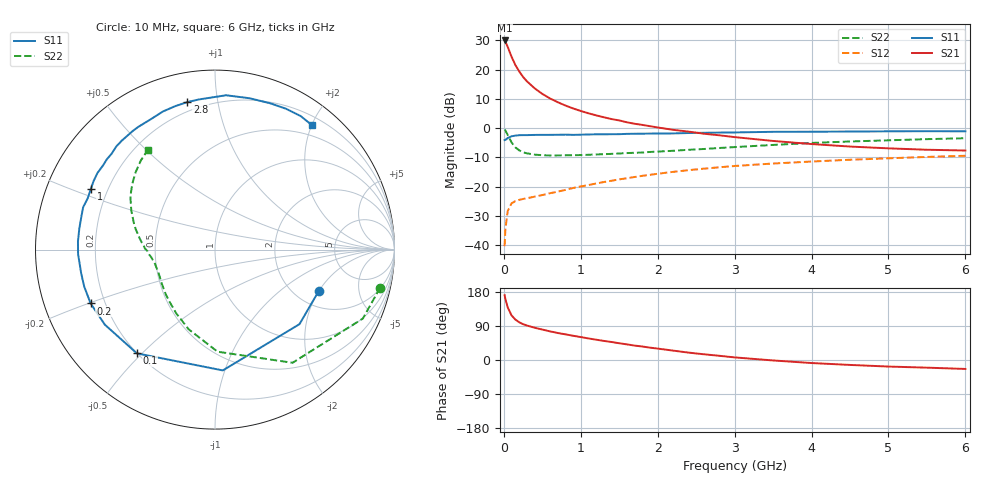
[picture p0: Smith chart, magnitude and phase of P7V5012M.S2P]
! SIEMENS Small Signal Semiconductors
! BFP196
! Si NPN RF Bipolar Junction Transistor in SOT143
! VCE = 0.5 V  IC = 12 mA
! Common Emitter S-Parameters:  May  1996
# GHz  S  MA  R  50
!  f  S11  S21  S12  S22
! GHz  MAG  ANG  MAG  ANG  MAG  ANG  MAG  ANG
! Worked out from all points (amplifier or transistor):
!   36 points, 10 MHz to 6 GHz, reference 50 ohm
!   highest |S21| = 29.9 dB at 10 MHz (marker M1)
!   |S21| within 3 dB of that: start of sweep to 62.4 MHz
!   unconditionally stable (mu >= 1): 744.5 MHz to end of sweep
!   at 250 MHz: K = 0.47, MSG = 20.8 dB, |S12| = -24.2 dB
!   at 1.4 GHz: K = 1.17, MAG = 8.0 dB, |S12| = -18.0 dB
!   at 6 GHz: K = 1.05, MAG = -0.5 dB, |S12| = -9.5 dB
!   S11 on the Smith chart (normalised r, x): 10 MHz: 2.66, -1.99; 100 MHz: 0.20, -0.48; 200 MHz: 0.15, -0.20; 1 GHz: 0.14, +0.23; 2.8 GHz: 0.15, +0.82; 6 GHz: 0.33, +2.01
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0.01  0.6227 -21.6  31.34 171.1  0.0096 81.4  0.944 -13.0
0.02  0.6278 -41.4  29.81 160.9  0.0186 71.0  0.909 -25.0
0.05  0.6746 -86.3  24.45 139.0  0.038 52.9  0.7643 -55.6
0.1  0.7236 -127.0  16.53 117.8  0.0517 37.2  0.569 -88.6
0.15  0.7426 -145.7  11.93 106.6  0.0566 30.6  0.4675 -108.3
0.2  0.7551 -156.6  9.261 99.6  0.0593 28.8  0.4153 -121.4
0.25  0.7572 -164.2  7.469 94.6  0.0615 28.1  0.3855 -131.1
0.3  0.7572 -169.8  6.287 91.0  0.0632 28.8  0.3702 -137.9
0.4  0.7632 -178.1  4.775 85.2  0.0673 30.4  0.3517 -147.6
0.5  0.7649 176.5  3.83 80.3  0.0716 32.4  0.3432 -153.7
0.6  0.765 171.0  3.205 75.6  0.077 34.8  0.3404 -158.1
0.7  0.7669 166.1  2.764 71.3  0.0819 36.8  0.341 -161.6
0.8  0.7716 162.2  2.425 67.7  0.0878 38.0  0.3421 -164.3
1  0.7701 153.8  1.957 60.5  0.1005 39.9  0.3455 -168.1
1.1  0.7767 150.6  1.786 56.9  0.1062 40.4  0.3496 -169.9
1.6  0.7954 133.8  1.254 41.2  0.139 40.2  0.3736 -177.3
2.2  0.8095 116.3  0.933 24.8  0.1784 35.7  0.4088 174.7
2.8  0.8363 100.6  0.752 11.1  0.2136 29.4  0.4565 165.5
3.5  0.8621 85.9  0.602 -1.2  0.2478 20.9  0.5146 155.0
4.5  0.8713 69.3  0.483 -13.0  0.2874 9.8  0.5894 141.4
5.5  0.8839 57.3  0.426 -20.2  0.3212 -0.6  0.6463 129.7
6  0.879 51.9  0.413 -23.6  0.3361 -6.3  0.67 123.9
